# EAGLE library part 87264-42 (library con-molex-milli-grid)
RECEPTACAL
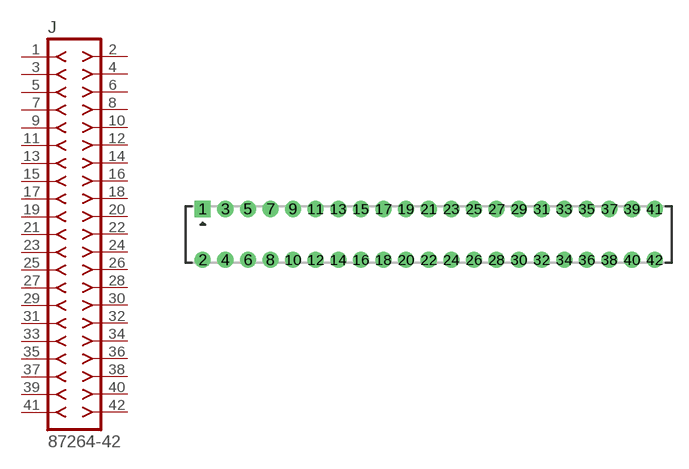
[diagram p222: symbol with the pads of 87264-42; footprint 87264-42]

Designator prefix J

## 87264-42  [87264-42]
1  1  pas
2  2  pas
3  3  pas
4  4  pas
5  5  pas
6  6  pas
7  7  pas
8  8  pas
9  9  pas
10  10  pas
11  11  pas
12  12  pas
13  13  pas
14  14  pas
15  15  pas
16  16  pas
17  17  pas
18  18  pas
19  19  pas
20  20  pas
21  21  pas
22  22  pas
23  23  pas
24  24  pas
25  25  pas
26  26  pas
27  27  pas
28  28  pas
29  29  pas
30  30  pas
31  31  pas
32  32  pas
33  33  pas
34  34  pas
35  35  pas
36  36  pas
37  37  pas
38  38  pas
39  39  pas
40  40  pas
41  41  pas
42  42  pas

## Footprint 87264-42 (pad centres in mm)
RECEPTACAL Dual Row, Side Entry
drill 0.914 square: 1 -20,2.25
drill 0.914: 2 -20,-2.25; 3 -18,2.25; 4 -18,-2.25; 5 -16,2.25; 6 -16,-2.25; 7 -14,2.25; 8 -14,-2.25; 9 -12,2.25; 10 -12,-2.25; 11 -10,2.25; 12 -10,-2.25; 13 -8,2.25; 14 -8,-2.25; 15 -6,2.25; 16 -6,-2.25; 17 -4,2.25; 18 -4,-2.25; 19 -2,2.25; 20 -2,-2.25; 21 0,2.25; 22 0,-2.25; 23 2,2.25; 24 2,-2.25; 25 4,2.25; 26 4,-2.25; 27 6,2.25; 28 6,-2.25; 29 8,2.25; 30 8,-2.25; 31 10,2.25; 32 10,-2.25; 33 12,2.25; 34 12,-2.25; 35 14,2.25; 36 14,-2.25; 37 16,2.25; 38 16,-2.25; 39 18,2.25; 40 18,-2.25; 41 20,2.25; 42 20,-2.25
